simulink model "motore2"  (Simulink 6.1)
settings: Solver=ode45  StartTime=0.0  StopTime=25  RelTol=1e-3
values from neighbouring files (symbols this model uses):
  B1 = 1.2    [Parametri.m]
  B2 = 2    [Parametri.m]
  B3 = 0.8    [Parametri.m]
  B4 = 0.4    [Parametri.m]
  Be = 0.1    [Parametri.m]
  bw1 = 0.03    [Parametri.m]
  bw2 = 0.15    [Parametri.m]
  bw3 = 0.15    [Parametri.m]
  bw4 = 0.15    [Parametri.m]
  Je = 0.15    [Parametri.m]
  Jw = Mv*R^2    (= 131.9486)    [Parametri.m]
  k1 = 40    [Parametri.m]
  k2 = 140    [Parametri.m]
  k3 = 180    [Parametri.m]
  k4 = 200    [Parametri.m]
  Mv = 1400    [Parametri.m]
  rw = R    (= 0.307)    [Parametri.m]
  tau1 = 0.0624    [Parametri.m]
  tau2 = 0.124    [Parametri.m]
  tau3 = 0.206    [Parametri.m]
  tau4 = 0.2795    [Parametri.m]
undefined symbols (not defined in the file or in its folder): MagicFormula
libraries: simulink x2

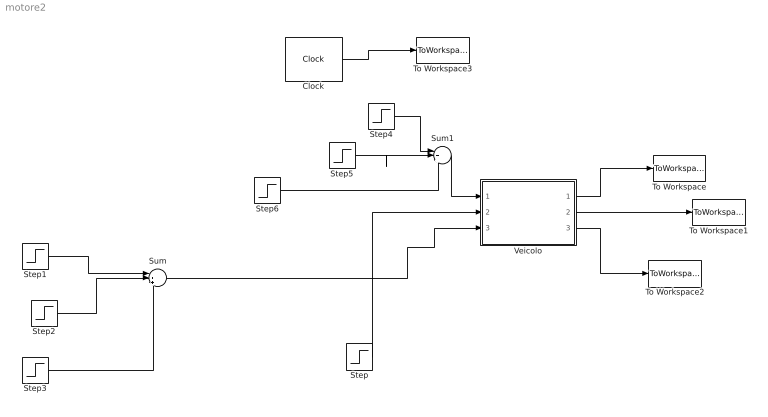
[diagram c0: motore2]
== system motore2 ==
  Clock : Clock
  Step : Step  After=150  SampleTime=0
  Step1 : Step  SampleTime=0
  Step2 : Step  Time=3  SampleTime=0
  Step3 : Step  Time=10  SampleTime=0
  Step4 : Step  Time=0  After=0.9  SampleTime=0
  Step5 : Step  Time=2  After=-0.4  SampleTime=0
  Step6 : Step  Time=4  After=+0.4  SampleTime=0
  Sum : Sum  Inputs=|+++
  Sum1 : Sum  Inputs=|+++
  To Workspace : ToWorkspace  VariableName=omegaw  SampleTime=-1  SaveFormat=Array
  To Workspace1 : ToWorkspace  VariableName=omegae  SampleTime=-1  SaveFormat=Array
  To Workspace2 : ToWorkspace  VariableName=v  SampleTime=-1  SaveFormat=Array
  To Workspace3 : ToWorkspace  VariableName=t  SampleTime=-1  SaveFormat=Array
  Veicolo : Subsystem
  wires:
  Sum/1 -> Veicolo/3(marcia corrente)
  Veicolo/1(omega_w) -> To Workspace/1
  Veicolo/2(omega_e) -> To Workspace1/1
  Veicolo/3(v_v) -> To Workspace2/1
  Clock/1 -> To Workspace3/1
  Step/1 -> Veicolo/2(accelleratore)
  Step1/1 -> Sum/1
  Step2/1 -> Sum/2
  Step3/1 -> Sum/3
  Sum1/1 -> Veicolo/1(mu)
  Step4/1 -> Sum1/1
  Step5/1 -> Sum1/2
  Step6/1 -> Sum1/3

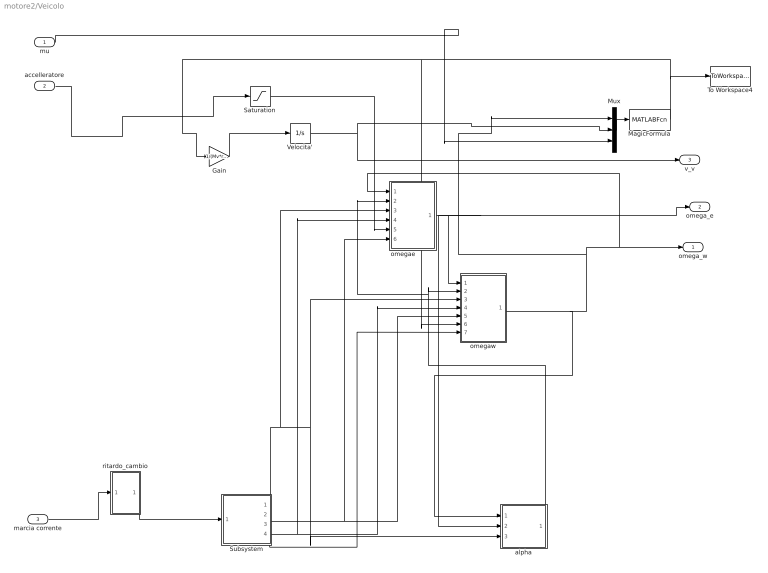
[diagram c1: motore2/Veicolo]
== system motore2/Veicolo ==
  mu : Inport  Port=1  LatchInput=off
  accelleratore : Inport  Port=2  LatchInput=off
  marcia corrente : Inport  Port=3  LatchInput=off
  Gain : Gain  Gain=1/(Mv*rw)
  MagicFormula : MATLABFcn  MATLABFcn=MagicFormula(u(1),u(2),u(3))  OutputDimensions=1
  Mux : Mux  Inputs=3
  Saturation : Saturate  UpperLimit=176  LowerLimit=-20
  Subsystem : Subsystem
  To Workspace4 : ToWorkspace  VariableName=Tw  SampleTime=-1  SaveFormat=Array
  Velocita' : Integrator  InitialCondition=0.1
  alpha : Subsystem
  omegae : Subsystem
  omegaw : Subsystem
  ritardo_cambio : Subsystem
  omega_w : Outport
  omega_e : Outport  Port=2
  v_v : Outport  Port=3
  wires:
  Gain/1 -> Velocita'/1
  Velocita'/1 -> v_v/1, Mux/2
  MagicFormula/1 -> omegaw/6(Tw), Gain/1, To Workspace4/1
  Subsystem/1(tau_i) -> alpha/3(taui), omegaw/3(taui), omegae/3(taui)
  Subsystem/2(b_i) -> omegaw/5(bi), omegae/6(bi)
  Subsystem/3(k_i) -> omegaw/4(ki), omegae/4(ki)
  alpha/1(alpha) -> omegaw/2(alpha), omegae/2(alpha)
  omegaw/1(omegaw) -> alpha/1(omegaw), omega_w/1, omegae/1(omegaw), Mux/1
  omegae/1(omegae) -> omegaw/1(omegae), omega_e/1, alpha/2(omegae)
  Subsystem/4(bw_i1) -> omegaw/7("bwi ")
  Mux/1 -> MagicFormula/1
  mu/1 -> Mux/3
  Saturation/1 -> omegae/5(Te)
  accelleratore/1 -> Saturation/1
  marcia corrente/1 -> ritardo_cambio/1(In1)
  ritardo_cambio/1(Out1) -> Subsystem/1(Marcia)

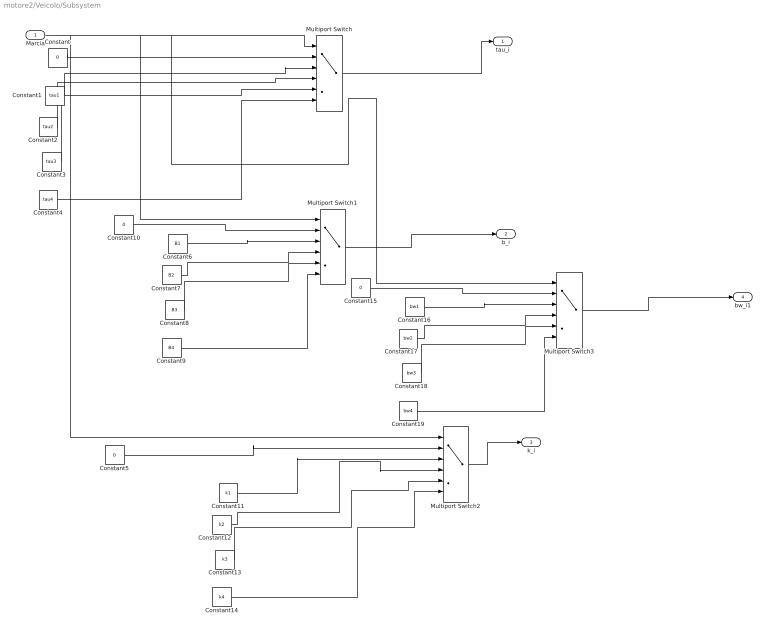
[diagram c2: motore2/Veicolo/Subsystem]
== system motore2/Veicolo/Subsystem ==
  Marcia : Inport  Port=1  LatchInput=off
  Constant{,5,10,15} (4 alike) : Constant  Value=0
  Constant1 : Constant  Value=tau1
  Constant11 : Constant  Value=k1
  Constant12 : Constant  Value=k2
  Constant13 : Constant  Value=k3
  Constant14 : Constant  Value=k4
  Constant16 : Constant  Value=bw1
  Constant17 : Constant  Value=bw2
  Constant18 : Constant  Value=bw3
  Constant19 : Constant  Value=bw4
  Constant2 : Constant  Value=tau2
  Constant3 : Constant  Value=tau3
  Constant4 : Constant  Value=tau4
  Constant6 : Constant  Value=B1
  Constant7 : Constant  Value=B2
  Constant8 : Constant  Value=B3
  Constant9 : Constant  Value=B4
  Multiport Switch{,1..3} (4 alike) : MultiPortSwitch  Inputs=5  zeroidx=on
  tau_i : Outport
  b_i : Outport  Port=2
  k_i : Outport  Port=3
  bw_i1 : Outport  Port=4
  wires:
  Marcia/1 -> Multiport Switch1/1, Multiport Switch/1, Multiport Switch3/1, Multiport Switch2/1
  Multiport Switch/1 -> tau_i/1
  Multiport Switch1/1 -> b_i/1
  Constant/1 -> Multiport Switch/2
  Constant1/1 -> Multiport Switch/3
  Constant2/1 -> Multiport Switch/4
  Constant3/1 -> Multiport Switch/5
  Constant4/1 -> Multiport Switch/6
  Constant5/1 -> Multiport Switch2/2
  Constant10/1 -> Multiport Switch1/2
  Constant6/1 -> Multiport Switch1/3
  Constant7/1 -> Multiport Switch1/4
  Constant8/1 -> Multiport Switch1/5
  Constant9/1 -> Multiport Switch1/6
  Constant11/1 -> Multiport Switch2/3
  Constant12/1 -> Multiport Switch2/4
  Constant13/1 -> Multiport Switch2/5
  Constant14/1 -> Multiport Switch2/6
  Multiport Switch2/1 -> k_i/1
  Multiport Switch3/1 -> bw_i1/1
  Constant15/1 -> Multiport Switch3/2
  Constant16/1 -> Multiport Switch3/3
  Constant17/1 -> Multiport Switch3/4
  Constant18/1 -> Multiport Switch3/5
  Constant19/1 -> Multiport Switch3/6

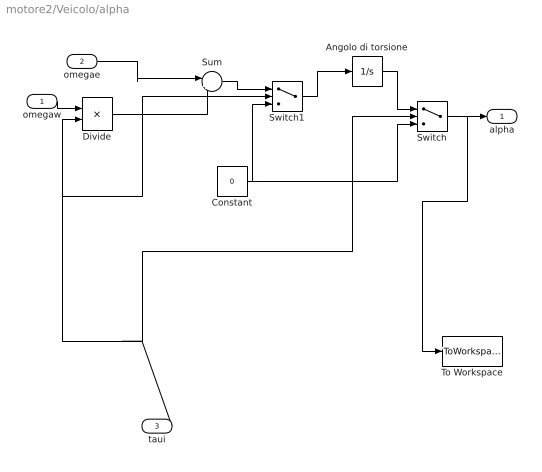
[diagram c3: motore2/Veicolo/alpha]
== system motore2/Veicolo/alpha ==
  omegaw : Inport  Port=1  LatchInput=off
  omegae : Inport  Port=2  LatchInput=off
  taui : Inport  Port=3  LatchInput=off
  Angolo di torsione : Integrator
  Constant : Constant  Value=0
  Divide : Product  Inputs=*/  OutScaling=2^-10
  Sum : Sum  Inputs=|+-
  Switch : Switch  Threshold=0.00001
  Switch1 : Switch  Threshold=0.00001
  To Workspace : ToWorkspace  VariableName=alpha  SampleTime=-1  SaveFormat=Array
  alpha : Outport
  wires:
  Angolo di torsione/1 -> Switch/1
  taui/1 -> Divide/2, Switch1/2, Switch/2
  Constant/1 -> Switch/3, Switch1/3
  Divide/1 -> Sum/2
  Switch/1 -> alpha/1, To Workspace/1
  omegaw/1 -> Divide/1
  omegae/1 -> Sum/1
  Switch1/1 -> Angolo di torsione/1
  Sum/1 -> Switch1/1

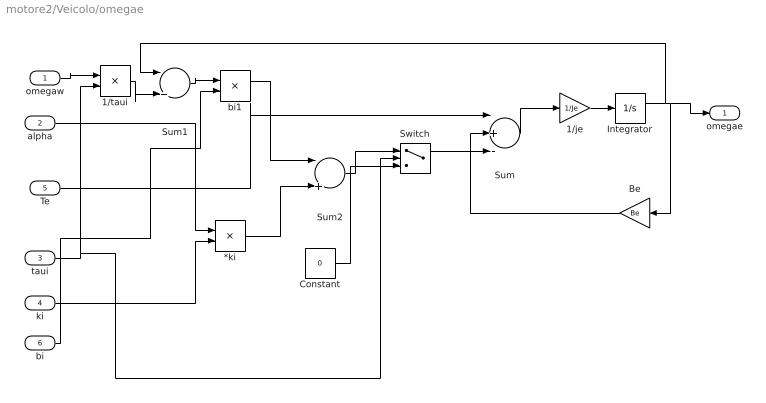
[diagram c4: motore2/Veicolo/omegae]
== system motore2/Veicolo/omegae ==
  omegaw : Inport  Port=1  LatchInput=off
  alpha : Inport  Port=2  LatchInput=off
  taui : Inport  Port=3  LatchInput=off
  ki : Inport  Port=4  LatchInput=off
  Te : Inport  Port=5  LatchInput=off
  bi : Inport  Port=6  LatchInput=off
  *ki : Product
  1/je : Gain  Gain=1/Je
  1/taui : Product  Inputs=*/  OutScaling=2^-10
  Be : Gain  Orientation=left  Gain=Be
  Constant : Constant  Value=0
  Integrator : Integrator
  Sum : Sum  Inputs=|+--
  Sum1 : Sum  Inputs=|+-
  Sum2 : Sum  Inputs=|++
  Switch : Switch  Threshold=0.00001
  bi1 : Product
  omegae : Outport
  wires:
  Integrator/1 -> omegae/1, Be/1, Sum1/1
  1/je/1 -> Integrator/1
  Sum/1 -> 1/je/1
  Be/1 -> Sum/2
  Te/1 -> Sum/1
  bi/1 -> bi1/2
  omegaw/1 -> 1/taui/1
  Sum1/1 -> bi1/1
  taui/1 -> 1/taui/2, Switch/2
  1/taui/1 -> Sum1/2
  ki/1 -> *ki/2
  alpha/1 -> *ki/1
  *ki/1 -> Sum2/2
  bi1/1 -> Sum2/1
  Switch/1 -> Sum/3
  Sum2/1 -> Switch/1
  Constant/1 -> Switch/3

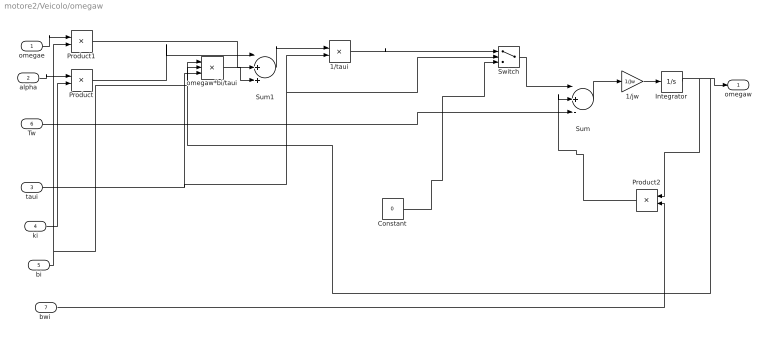
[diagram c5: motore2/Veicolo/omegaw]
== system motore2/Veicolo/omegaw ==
  omegae : Inport  Port=1  LatchInput=off
  alpha : Inport  Port=2  LatchInput=off
  taui : Inport  Port=3  LatchInput=off
  ki : Inport  Port=4  LatchInput=off
  bi : Inport  Port=5  LatchInput=off
  Tw : Inport  Port=6  LatchInput=off
  "bwi " : Inport  Port=7  LatchInput=off
  1/jw : Gain  Gain=1/Jw
  1/taui : Product  Inputs=*/  OutScaling=2^-10
  Constant : Constant  Value=0
  Integrator : Integrator
  Product : Product
  Product1 : Product
  Product2 : Product  Orientation=left
  Sum : Sum  Inputs=|+--
  Sum1 : Sum  Inputs=|++-
  Switch : Switch  Threshold=0.00001
  omegaw*bi/taui : Product  Inputs=**/  OutScaling=2^-10
  omegaw : Outport
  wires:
  Integrator/1 -> omegaw/1, omegaw*bi/taui/1, Product2/1
  1/jw/1 -> Integrator/1
  Sum/1 -> 1/jw/1
  Product2/1 -> Sum/2
  Tw/1 -> Sum/3
  alpha/1 -> Product/1
  ki/1 -> Product/2
  Sum1/1 -> 1/taui/1
  Product/1 -> Sum1/1
  taui/1 -> omegaw*bi/taui/3, 1/taui/2, Switch/2
  omegae/1 -> Product1/1
  bi/1 -> Product1/2, omegaw*bi/taui/2
  Product1/1 -> Sum1/2
  omegaw*bi/taui/1 -> Sum1/3
  "bwi "/1 -> Product2/2
  Switch/1 -> Sum/1
  1/taui/1 -> Switch/1
  Constant/1 -> Switch/3

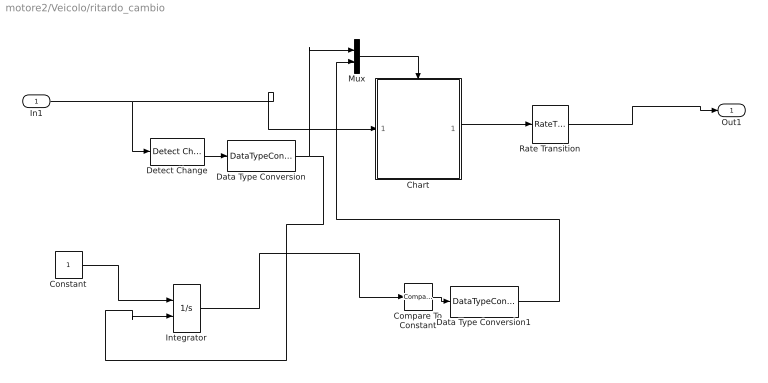
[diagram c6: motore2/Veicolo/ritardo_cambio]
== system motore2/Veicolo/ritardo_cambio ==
  In1 : Inport  Port=1  LatchInput=off
  Chart : Stateflow chart
  Compare To Constant : simulink/Logic and Bit Operations/Compare To Constant  relop=>=  const=1e-1  LogicOutDataTypeMode=uint8  ZeroCross=off
  Constant : Constant
  Data Type Conversion : DataTypeConversion
  Data Type Conversion1 : DataTypeConversion
  Detect Change : simulink/Logic and Bit Operations/Detect Change  vinit=0
  Integrator : Integrator  ExternalReset=either
  Mux : Mux  Inputs=2
  Rate Transition : RateTransition  OutPortSampleTime=0
  Out1 : Outport
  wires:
  Chart/1(marcia_out) -> Rate Transition/1
  Rate Transition/1 -> Out1/1
  In1/1 -> Chart/1(marcia), Detect Change/1
  Detect Change/1 -> Data Type Conversion/1
  Integrator/1 -> Compare To Constant/1
  Data Type Conversion/1 -> Integrator/2, Mux/1
  Constant/1 -> Integrator/1
  Mux/1 -> Chart/Trigger
  Compare To Constant/1 -> Data Type Conversion1/1
  Data Type Conversion1/1 -> Mux/2

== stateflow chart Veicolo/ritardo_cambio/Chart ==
  state s0
    en: marcia_out = marcia;
  state s1
    en:marcia_out = 0;
  (default) -> s0
  s0 -> s1 : trigger
  s1 -> s0 : CLK_EXPIRE
